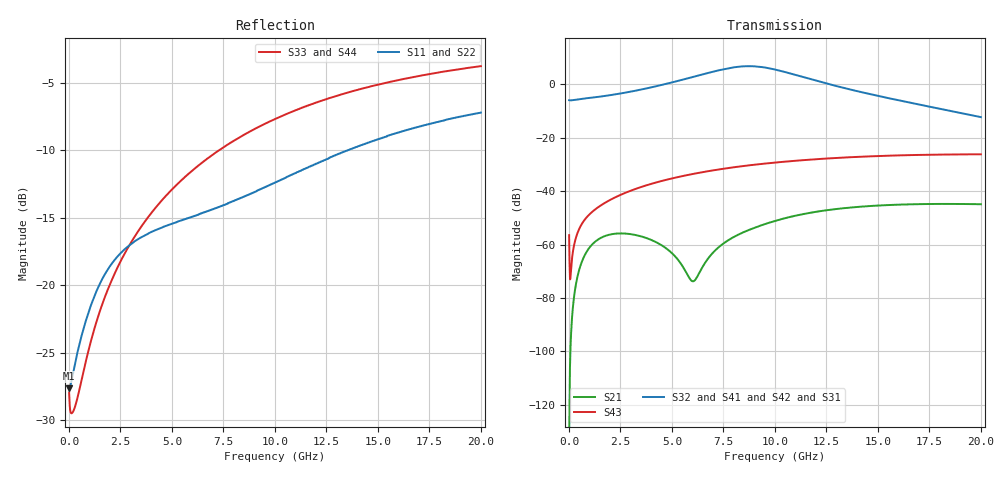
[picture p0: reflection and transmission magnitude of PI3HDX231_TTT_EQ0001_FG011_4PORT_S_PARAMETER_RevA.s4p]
! NPort=4 DATA=2000 NOISE=0 GROUPDELAY=0 COMPLEX_DATAFORMAT=POLAR
! NumOfBlock=1 NumOfParam=0
! .MODEL Smodel S TSTONEFILE=PI3HDX231_TTT_EQ0001_FG011_4PORT_S_PARAMETER_RevA.s4p TYPE=S
!  -- The above .MODEL line can be used for the S element in the netlist.
! The s parameter is extracted from the linear redriver, it is not bi-directional; only s(4,1)s(4,2) and s(3,1)s(3,2)
! should be the insertion loss
!Port definition:
!Port1 = input+
!Port2 = input-
!Port3 = output+
!Port4 = output-
# Hz S MA R  50
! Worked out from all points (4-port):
!   2000 points, 10 MHz to 20 GHz, reference 50 ohm
!   strongest paths, dB at 10 MHz, 5.01 GHz, 10.01 GHz, 15.01 GHz, 20 GHz:
!     S32: -5.9, 0.7, 5.5, -4.3, -12.3
!     S41: -5.9, 0.8, 5.5, -4.4, -12.4
!     S42: -5.9, 0.8, 5.5, -4.4, -12.1
!     S31: -5.9, 0.7, 5.3, -4.7, -12.5
!     S43: -56.5, -35.2, -29.3, -26.9, -26.2
!     S21: -134.8, -63.3, -51.1, -45.4, -44.9
!   lowest |S11| = -27.6 dB at 10 MHz (marker M1), VSWR 1.09, Z = 46 - j0.0776 ohm
!   |S11| at or under -10 dB: start of sweep to 13.55 GHz
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1e7  0.04152 -178.8  1.825e-07 -14.0  0 0.0  0 0.0
     1.825e-07 -13.9  0.04152 -178.8  0 0.0  0 0.0
     0.5041 -0.7  0.5041 179.3  0.04012 -3.2  0.0015 -70.3
     0.5041 179.3  0.5041 -0.7  0.0015 -70.3  0.04012 -3.2
2.09e9  0.1205 -139.6  0.001566 42.1  2.308e-12 -68.7  2.071e-12 -59.3
        0.001566 42.1  0.1205 -139.6  2.019e-12 -60.7  2.365e-12 -67.2
        0.6249 -11.7  0.6342 168.5  0.105 -90.3  0.007141 73.6
        0.6359 168.7  0.625 -10.8  0.00714 73.6  0.105 -90.2
5.8e9  0.1772 -138.7  0.0002492 8.6  1.335e-09 168.8  5.534e-10 -159.6
       0.0002534 10.0  0.1771 -138.9  5.149e-10 -158.1  1.416e-09 168.7
       1.301 -63.2  1.304 116.1  0.258 -104.8  0.02025 57.1
       1.308 115.8  1.326 -61.8  0.02019 57.1  0.2581 -104.8
7.77e9  0.2019 -134.0  0.001226 100.5  8.744e-09 105.7  3.398e-09 -179.6
        0.001229 99.8  0.2013 -134.2  3.29e-09 -176.1  9.299e-09 104.2
        1.992 -117.0  2.008 62.4  0.3339 -110.1  0.02729 45.0
        2.008 62.1  2.038 -115.7  0.02719 45.0  0.334 -110.1
9.24e9  0.2257 -130.8  0.002228 89.1  2.223e-08 54.6  1.405e-08 138.4
        0.002223 88.6  0.2247 -131.0  1.379e-08 141.2  2.35e-08 52.1
        2.095 -172.0  2.134 7.4  0.3865 -113.8  0.03209 35.4
        2.129 7.0  2.147 -170.7  0.03197 35.5  0.3866 -113.9
1.138e10  0.2679 -128.3  0.003737 68.6  5.133e-08 -1.0  4.533e-08 63.2
          0.003722 68.2  0.2663 -128.5  4.473e-08 65.7  5.308e-08 -4.3
          1.318 121.7  1.365 -59.7  0.4555 -118.9  0.03816 21.5
          1.357 -60.0  1.353 123.2  0.03806 21.6  0.4555 -118.9
2e10  0.4354 -135.6  0.00572 -4.9  3.771e-07 -160.0  2.781e-07 -129.5
      0.005686 -5.0  0.4337 -135.4  2.788e-07 -128.0  3.717e-07 -162.8
      0.2359 -24.4  0.2431 148.5  0.6464 -135.0  0.04881 -32.2
      0.2411 149.0  0.2486 -22.7  0.04894 -32.0  0.6461 -135.0
